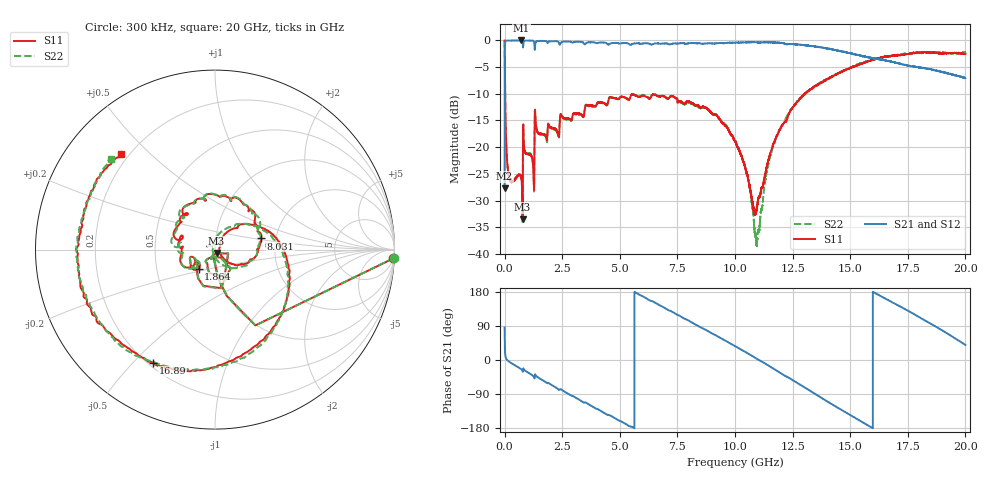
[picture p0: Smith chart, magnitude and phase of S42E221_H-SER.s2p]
! Created Wed Nov 25 22:05:23 2020
# khz S ma R 50
! 2 Port Network Data from SP1.SP block
! freq  magS11  angS11  magS21  angS21  magS12  angS12  magS22  angS22
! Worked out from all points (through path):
!   20001 points, 300 kHz to 20 GHz, reference 50 ohm
!   highest |S21| = -0.02 dB at 721.3 MHz (marker M1); lowest = -27.7 dB at 300 kHz (marker M2)
!   group delay of S21, straight-line fit = 94.7 ps
!   lowest |S11| = -33.5 dB at 781.3 MHz (marker M3), VSWR 1.04, Z = 50.8 - j1.97 ohm
!   |S11| at or under -10 dB: 21.82 MHz to 13.02 GHz (13 GHz wide, 199 % of centre); 13.02343 GHz to 13.02662 GHz (3.193 MHz wide, 0.0245 % of centre); 13.02788 GHz to 13.02883 GHz (947.1 kHz wide, 0.00727 % of centre)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
!   |S22| runs from -38.5 to 0.0 dB; largest |S21 - S12| = 0.019
!   S11 on the Smith chart (normalised r, x): 300 kHz: 4, -41; 1.864 GHz: 0.82, -0.18; 8.031 GHz: 1.68, +0.23; 16.89 GHz: 0.22, -0.57; 20 GHz: 0.17, +0.41
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300  0.9956 -2.8  0.04136 85.7  0.04151 86.8  0.9985 -2.7
102300  0.07813 -90.4  0.9954 0.6  0.9956 0.6  0.07887 -90.4
195300  0.05206 -96.7  0.9963 -4.4  0.9966 -4.4  0.05255 -97.0
721300  0.05188 -113.7  0.9982 -24.2  0.9976 -24.2  0.05229 -116.1
781300  0.02115 -66.7  0.9831 -28.6  0.9823 -28.6  0.01939 -73.4
1197300  0.07832 -129.6  0.9937 -40.2  0.9926 -40.1  0.07982 -130.0
1398300  0.1437 -133.3  0.9837 -43.6  0.9836 -43.6  0.1459 -131.8
1864300  0.1411 -130.2  0.9425 -60.9  0.9424 -61.0  0.1344 -133.5
3334300  0.2022 157.2  0.9674 -108.4  0.9677 -108.4  0.199 168.2
5198300  0.2935 103.5  0.9438 -166.8  0.9447 -166.8  0.2922 104.3
6667300  0.2988 58.5  0.9382 146.3  0.9353 146.3  0.3013 57.9
8031300  0.2655 13.6  0.9421 102.4  0.9401 102.7  0.261 13.1
1.00003e7  0.1141 -41.9  0.9507 36.7  0.953 36.8  0.1155 -55.8
1.04993e7  0.05817 -45.3  0.9585 19.4  0.9584 19.4  0.05813 -81.4
1.09563e7  0.02744 23.8  0.9589 2.8  0.9601 2.8  0.01238 143.8
1.17263e7  0.1146 55.7  0.9546 -24.9  0.9548 -24.8  0.1112 68.6
1.33343e7  0.3546 8.1  0.8838 -84.1  0.8857 -83.8  0.3575 3.3
1.50333e7  0.5565 -57.4  0.7532 -146.3  0.7554 -146.5  0.5597 -56.0
1.66673e7  0.7084 -111.5  0.6416 157.7  0.6276 157.8  0.7045 -113.1
1.68933e7  0.7204 -118.7  0.6256 150.2  0.6134 150.4  0.7173 -120.0
1.83293e7  0.7727 -168.6  0.5433 101.6  0.5468 102.4  0.7657 -164.0
2e7  0.7483 134.5  0.4431 39.9  0.4465 40.9  0.7651 138.9
